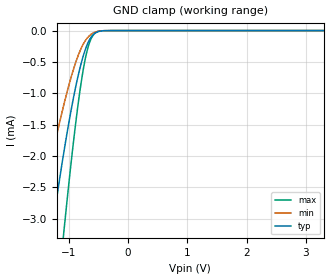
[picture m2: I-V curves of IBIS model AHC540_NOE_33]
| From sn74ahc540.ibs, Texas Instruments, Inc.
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[Model]   AHC540_NOE_33
Model_type  Input
Vinl = 0.9
Vinh = 2.1
| variable   typ   min   max
C_comp   0.67pF   0.59pF   0.76pF
[Temperature Range]   40   100   -40
| Ambient temperature   25   85   -40
[Voltage range]   3.3   3   3.6
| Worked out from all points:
|   GND clamp passes 1 mA (typ) near -0.91 V on its own axis
[GND Clamp]
| AHC540_NOE_33
|   Voltage   I(typ)   I(min)   I(max)
-5V       -39.52mA   -26.01mA   -50.56mA
-1.55V    -5.112mA   -3.269mA   -8.044mA
-1.5V     -4.736mA   -3.022mA   -7.496mA
-1.295V   -3.277mA   -2.064mA   -5.315mA
-1.245V   -2.945mA   -1.845mA   -4.803mA
-1.08V    -1.924mA   -1.171mA   -3.185mA
-910mV    -1.023mA   -586.6uA   -1.69mA
-785mV    -503uA     -271.8uA   -792.8uA
-680mV    -204.3uA   -109.6uA   -284uA
-630mV    -114.3uA   -64.05uA   -144.4uA
-555mV    -38.58uA   -24.2uA    -40.51uA
3.3V      3.885nA    645.3pA    18.64nA
